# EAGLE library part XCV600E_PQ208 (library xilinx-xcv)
xcv600e_pq208 edit this description Auto generated by make-symbol-device-package-bsdl.ulp Rev. 26 Source: xcv600e_pq208.bsd
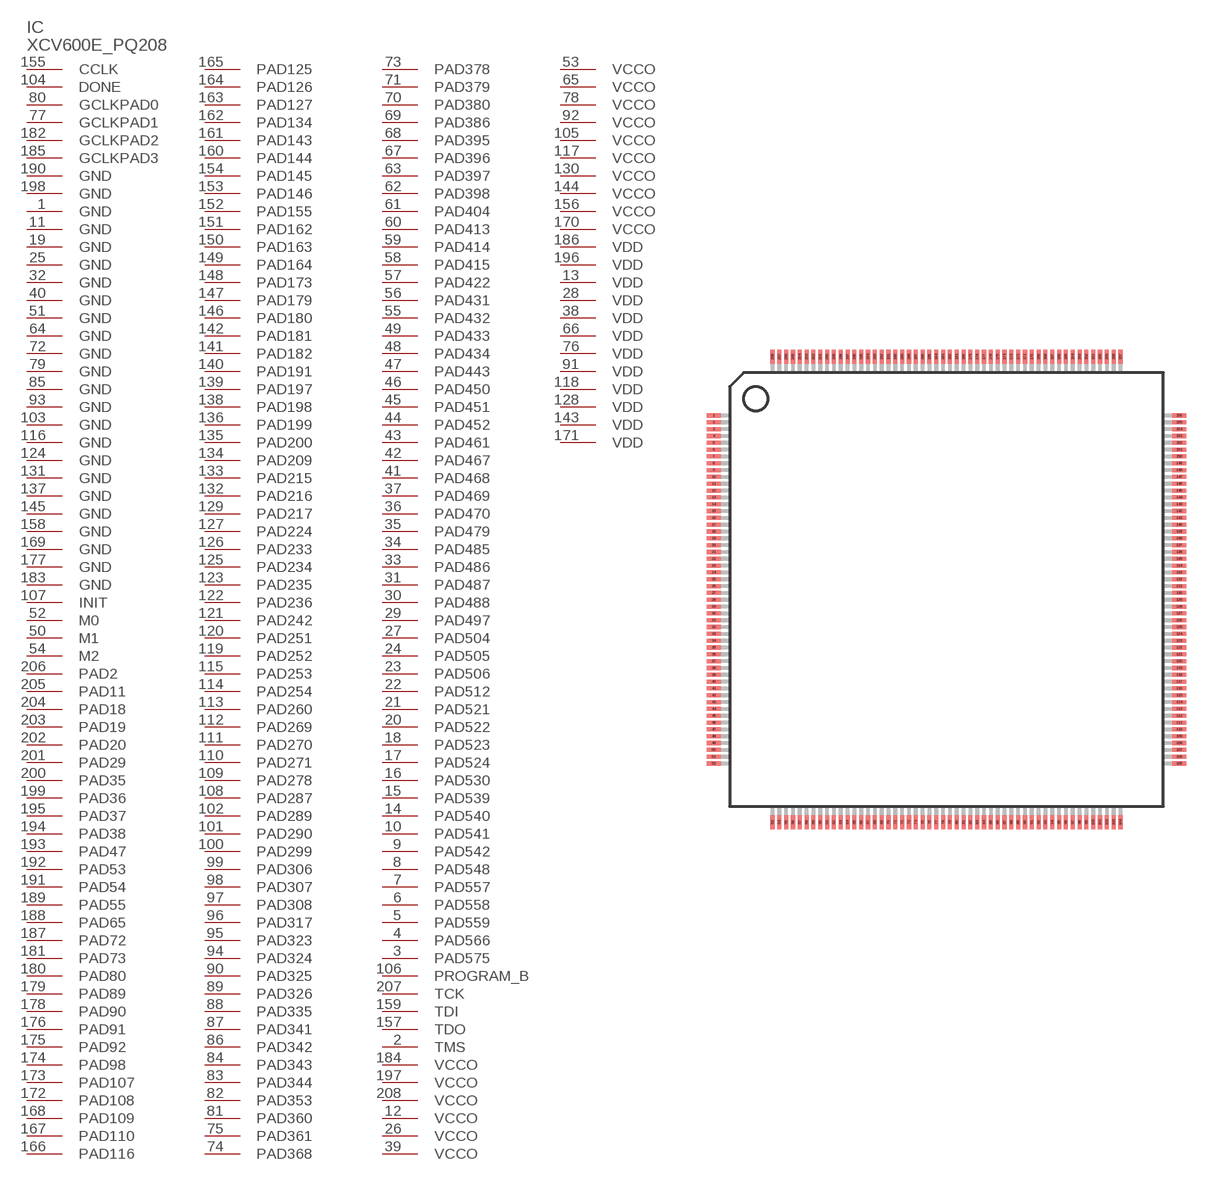
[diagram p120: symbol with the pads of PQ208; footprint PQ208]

Designator prefix IC

## XCV600E_PQ208 (OC_FARNELL: unknown; OC_NEWARK: unknown)  [PQ208]
1  GND  pwr
2  TMS  in
3  PAD575
4  PAD566
5  PAD559
6  PAD558
7  PAD557
8  PAD548
9  PAD542
10  PAD541
11  GND  pwr
12  VCCO  pwr
13  VDD  pwr
14  PAD540
15  PAD539
16  PAD530
17  PAD524
18  PAD523
19  GND  pwr
20  PAD522
21  PAD521
22  PAD512
23  PAD506
24  PAD505
25  GND  pwr
26  VCCO  pwr
27  PAD504
28  VDD  pwr
29  PAD497
30  PAD488
31  PAD487
32  GND  pwr
33  PAD486
34  PAD485
35  PAD479
36  PAD470
37  PAD469
38  VDD  pwr
39  VCCO  pwr
40  GND  pwr
41  PAD468
42  PAD467
43  PAD461
44  PAD452
45  PAD451
46  PAD450
47  PAD443
48  PAD434
49  PAD433
50  M1  in
51  GND  pwr
52  M0  in
53  VCCO  pwr
54  M2  in
55  PAD432
56  PAD431
57  PAD422
58  PAD415
59  PAD414
60  PAD413
61  PAD404
62  PAD398
63  PAD397
64  GND  pwr
65  VCCO  pwr
66  VDD  pwr
67  PAD396
68  PAD395
69  PAD386
70  PAD380
71  PAD379
72  GND  pwr
73  PAD378
74  PAD368
75  PAD361
76  VDD  pwr
77  GCLKPAD1  in
78  VCCO  pwr
79  GND  pwr
80  GCLKPAD0  in
81  PAD360
82  PAD353
83  PAD344
84  PAD343
85  GND  pwr
86  PAD342
87  PAD341
88  PAD335
89  PAD326
90  PAD325
91  VDD  pwr
92  VCCO  pwr
93  GND  pwr
94  PAD324
95  PAD323
96  PAD317
97  PAD308
98  PAD307
99  PAD306
100  PAD299
101  PAD290
102  PAD289
103  GND  pwr
104  DONE
105  VCCO  pwr
106  PROGRAM_B  in
107  INIT
108  PAD287
109  PAD278
110  PAD271
111  PAD270
112  PAD269
113  PAD260
114  PAD254
115  PAD253
116  GND  pwr
117  VCCO  pwr
118  VDD  pwr
119  PAD252
120  PAD251
121  PAD242
122  PAD236
123  PAD235
124  GND  pwr
125  PAD234
126  PAD233
127  PAD224
128  VDD  pwr
129  PAD217
130  VCCO  pwr
131  GND  pwr
132  PAD216
133  PAD215
134  PAD209
135  PAD200
136  PAD199
137  GND  pwr
138  PAD198
139  PAD197
140  PAD191
141  PAD182
142  PAD181
143  VDD  pwr
144  VCCO  pwr
145  GND  pwr
146  PAD180
147  PAD179
148  PAD173
149  PAD164
150  PAD163
151  PAD162
152  PAD155
153  PAD146
154  PAD145
155  CCLK
156  VCCO  pwr
157  TDO  out
158  GND  pwr
159  TDI  in
160  PAD144
161  PAD143
162  PAD134
163  PAD127
164  PAD126
165  PAD125
166  PAD116
167  PAD110
168  PAD109
169  GND  pwr
170  VCCO  pwr
171  VDD  pwr
172  PAD108
173  PAD107
174  PAD98
175  PAD92
176  PAD91
177  GND  pwr
178  PAD90
179  PAD89
180  PAD80
181  PAD73
182  GCLKPAD2  in
183  GND  pwr
184  VCCO  pwr
185  GCLKPAD3  in
186  VDD  pwr
187  PAD72
188  PAD65
189  PAD55
190  GND  pwr
191  PAD54
192  PAD53
193  PAD47
194  PAD38
195  PAD37
196  VDD  pwr
197  VCCO  pwr
198  GND  pwr
199  PAD36
200  PAD35
201  PAD29
202  PAD20
203  PAD19
204  PAD18
205  PAD11
206  PAD2
207  TCK  in
208  VCCO  pwr

## Footprint PQ208 (pad centres in mm)
PQ208 Auto generated by make-symbol-device-package-bsdl.ulp Rev. 26
smd 1 x 0.3: 1 -17.05,12.75; 2 -17.05,12.25; 3 -17.05,11.75; 4 -17.05,11.25; 5 -17.05,10.75; 6 -17.05,10.25; 7 -17.05,9.75; 8 -17.05,9.25; 9 -17.05,8.75; 10 -17.05,8.25; 11 -17.05,7.75; 12 -17.05,7.25; 13 -17.05,6.75; 14 -17.05,6.25; 15 -17.05,5.75; 16 -17.05,5.25; 17 -17.05,4.75; 18 -17.05,4.25; 19 -17.05,3.75; 20 -17.05,3.25; 21 -17.05,2.75; 22 -17.05,2.25; 23 -17.05,1.75; 24 -17.05,1.25; 25 -17.05,0.75; 26 -17.05,0.25; 27 -17.05,-0.25; 28 -17.05,-0.75; 29 -17.05,-1.25; 30 -17.05,-1.75; 31 -17.05,-2.25; 32 -17.05,-2.75; 33 -17.05,-3.25; 34 -17.05,-3.75; 35 -17.05,-4.25; 36 -17.05,-4.75; 37 -17.05,-5.25; 38 -17.05,-5.75; 39 -17.05,-6.25; 40 -17.05,-6.75; 41 -17.05,-7.25; 42 -17.05,-7.75; 43 -17.05,-8.25; 44 -17.05,-8.75; 45 -17.05,-9.25; 46 -17.05,-9.75; 47 -17.05,-10.25; 48 -17.05,-10.75; 49 -17.05,-11.25; 50 -17.05,-11.75; 51 -17.05,-12.25; 52 -17.05,-12.75; 105 17.05,-12.75; 106 17.05,-12.25; 107 17.05,-11.75; 108 17.05,-11.25; 109 17.05,-10.75; 110 17.05,-10.25; 111 17.05,-9.75; 112 17.05,-9.25; 113 17.05,-8.75; 114 17.05,-8.25; 115 17.05,-7.75; 116 17.05,-7.25; 117 17.05,-6.75; 118 17.05,-6.25; 119 17.05,-5.75; 120 17.05,-5.25; 121 17.05,-4.75; 122 17.05,-4.25; 123 17.05,-3.75; 124 17.05,-3.25; 125 17.05,-2.75; 126 17.05,-2.25; 127 17.05,-1.75; 128 17.05,-1.25; 129 17.05,-0.75; 130 17.05,-0.25; 131 17.05,0.25; 132 17.05,0.75; 133 17.05,1.25; 134 17.05,1.75; 135 17.05,2.25; 136 17.05,2.75; 137 17.05,3.25; 138 17.05,3.75; 139 17.05,4.25; 140 17.05,4.75; 141 17.05,5.25; 142 17.05,5.75; 143 17.05,6.25; 144 17.05,6.75; 145 17.05,7.25; 146 17.05,7.75; 147 17.05,8.25; 148 17.05,8.75; 149 17.05,9.25; 150 17.05,9.75; 151 17.05,10.25; 152 17.05,10.75; 153 17.05,11.25; 154 17.05,11.75; 155 17.05,12.25; 156 17.05,12.75
smd 0.3 x 1: 53 -12.75,-17.05; 54 -12.25,-17.05; 55 -11.75,-17.05; 56 -11.25,-17.05; 57 -10.75,-17.05; 58 -10.25,-17.05; 59 -9.75,-17.05; 60 -9.25,-17.05; 61 -8.75,-17.05; 62 -8.25,-17.05; 63 -7.75,-17.05; 64 -7.25,-17.05; 65 -6.75,-17.05; 66 -6.25,-17.05; 67 -5.75,-17.05; 68 -5.25,-17.05; 69 -4.75,-17.05; 70 -4.25,-17.05; 71 -3.75,-17.05; 72 -3.25,-17.05; 73 -2.75,-17.05; 74 -2.25,-17.05; 75 -1.75,-17.05; 76 -1.25,-17.05; 77 -0.75,-17.05; 78 -0.25,-17.05; 79 0.25,-17.05; 80 0.75,-17.05; 81 1.25,-17.05; 82 1.75,-17.05; 83 2.25,-17.05; 84 2.75,-17.05; 85 3.25,-17.05; 86 3.75,-17.05; 87 4.25,-17.05; 88 4.75,-17.05; 89 5.25,-17.05; 90 5.75,-17.05; 91 6.25,-17.05; 92 6.75,-17.05; 93 7.25,-17.05; 94 7.75,-17.05; 95 8.25,-17.05; 96 8.75,-17.05; 97 9.25,-17.05; 98 9.75,-17.05; 99 10.25,-17.05; 100 10.75,-17.05; 101 11.25,-17.05; 102 11.75,-17.05; 103 12.25,-17.05; 104 12.75,-17.05; 157 12.75,17.05; 158 12.25,17.05; 159 11.75,17.05; 160 11.25,17.05; 161 10.75,17.05; 162 10.25,17.05; 163 9.75,17.05; 164 9.25,17.05; 165 8.75,17.05; 166 8.25,17.05; 167 7.75,17.05; 168 7.25,17.05; 169 6.75,17.05; 170 6.25,17.05; 171 5.75,17.05; 172 5.25,17.05; 173 4.75,17.05; 174 4.25,17.05; 175 3.75,17.05; 176 3.25,17.05; 177 2.75,17.05; 178 2.25,17.05; 179 1.75,17.05; 180 1.25,17.05; 181 0.75,17.05; 182 0.25,17.05; 183 -0.25,17.05; 184 -0.75,17.05; 185 -1.25,17.05; 186 -1.75,17.05; 187 -2.25,17.05; 188 -2.75,17.05; 189 -3.25,17.05; 190 -3.75,17.05; 191 -4.25,17.05; 192 -4.75,17.05; 193 -5.25,17.05; 194 -5.75,17.05; 195 -6.25,17.05; 196 -6.75,17.05; 197 -7.25,17.05; 198 -7.75,17.05; 199 -8.25,17.05; 200 -8.75,17.05; 201 -9.25,17.05; 202 -9.75,17.05; 203 -10.25,17.05; 204 -10.75,17.05; 205 -11.25,17.05; 206 -11.75,17.05; 207 -12.25,17.05; 208 -12.75,17.05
